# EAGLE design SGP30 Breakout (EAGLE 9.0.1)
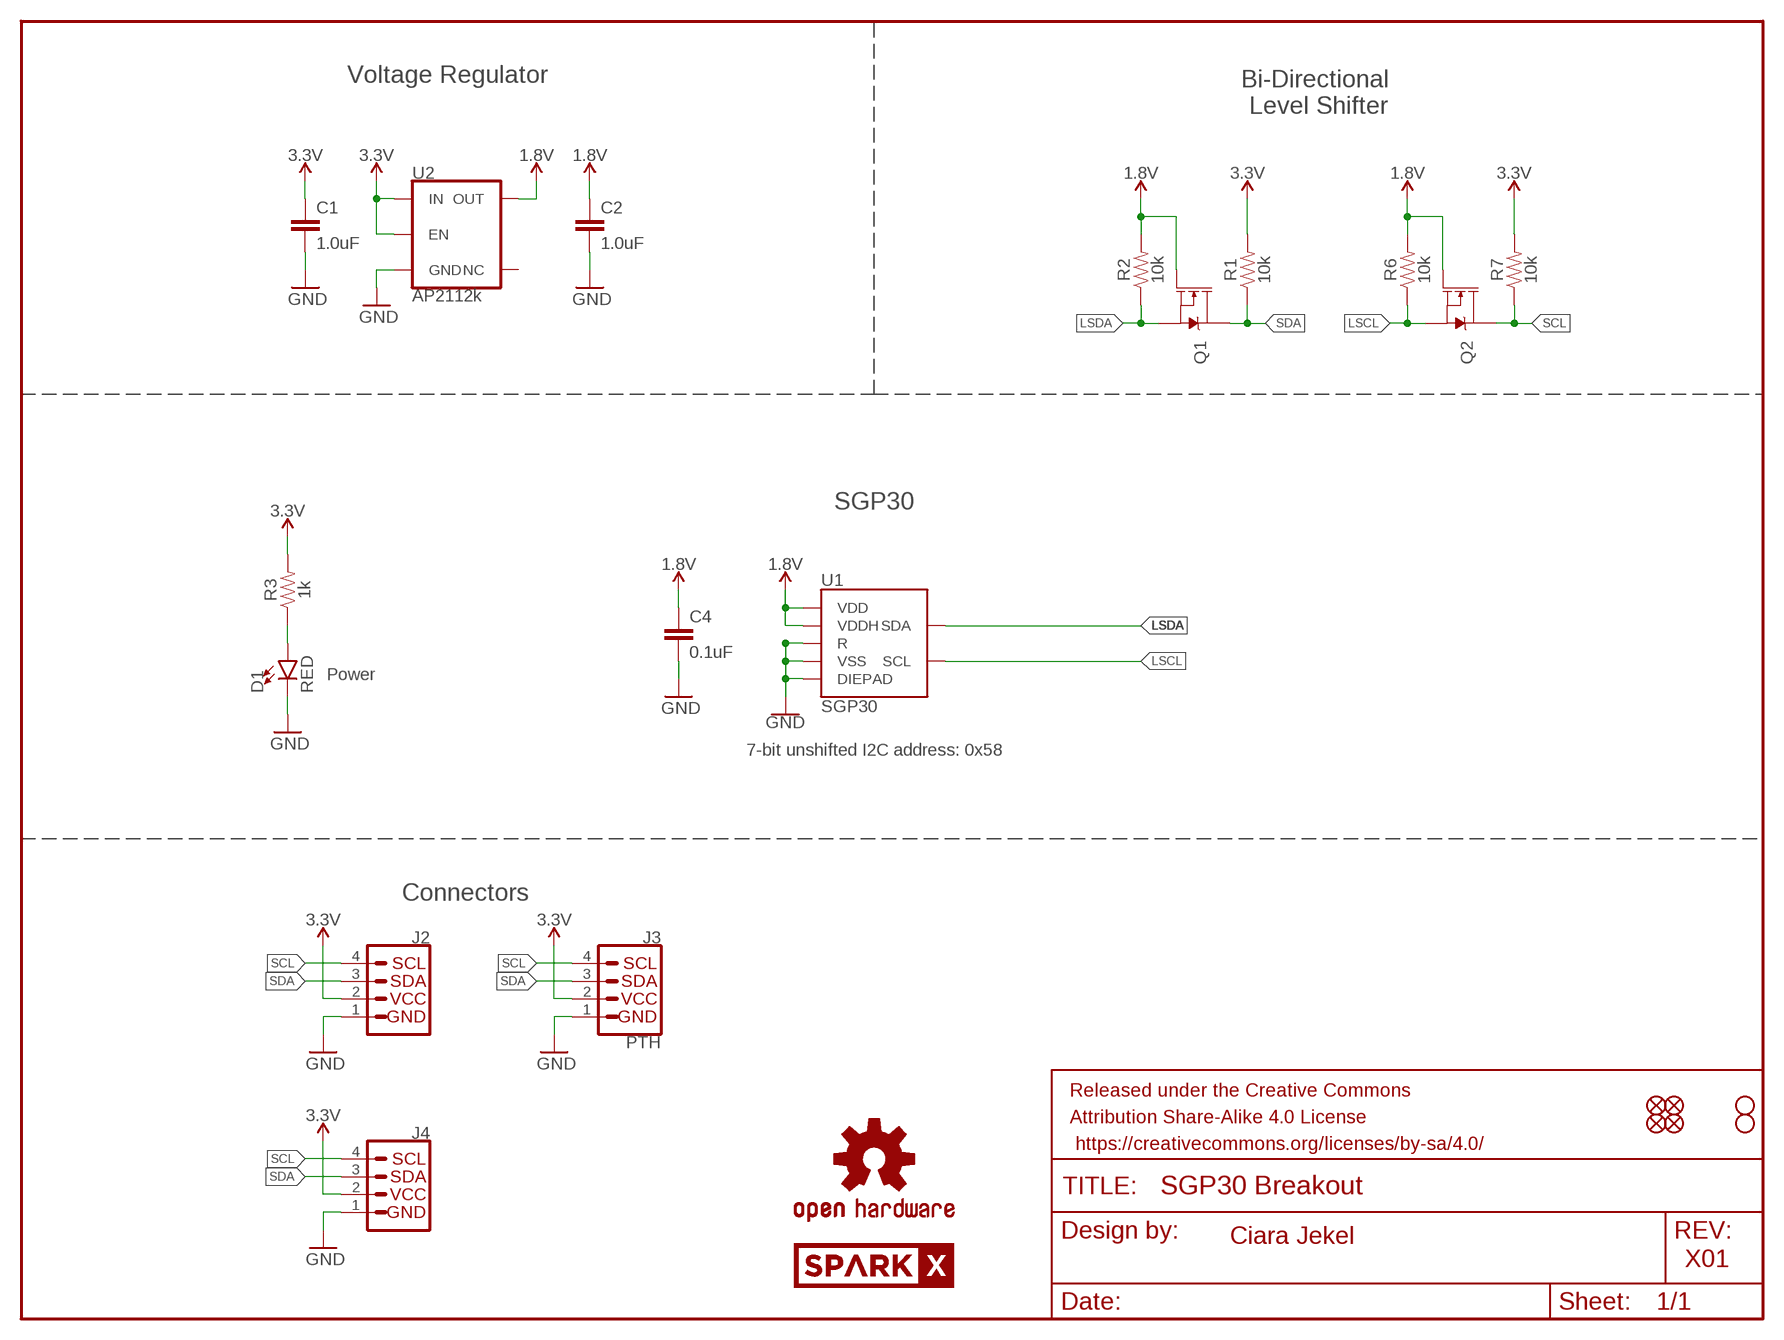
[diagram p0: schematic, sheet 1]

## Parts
C1  1.0uF  1.0UF-0603-16V-10%  [0603]
C2  1.0uF  1.0UF-0603-16V-10%  [0603]
C4  0.1uF  0.1UF-0603-25V-(+80/-20%)  [0603]
D1  RED  LED-RED0603  [LED-0603]
FRAME1  FRAME-LETTER  [CREATIVE_COMMONS]
J2  QWIIC_CONNECTORJS-1MM  [1X04_1MM_RA]
J3  PTH  I2C_STANDARD_NO_SILK  [1X04_NO_SILK]
J4  QWIIC_CONNECTORJS-1MM  [1X04_1MM_RA]
JP1  FIDUCIALUFIDUCIAL  [MICRO-FIDUCIAL]
JP2  FIDUCIALUFIDUCIAL  [MICRO-FIDUCIAL]
JP3  STAND-OFF  [STAND-OFF]
JP4  STAND-OFF  [STAND-OFF]
JP5  FIDUCIALUFIDUCIAL  [MICRO-FIDUCIAL]
JP6  FIDUCIALUFIDUCIAL  [MICRO-FIDUCIAL]
LOGO1  OSHW-LOGOMINI  [OSHW-LOGO-MINI]
Q1  MOSFET-NCH-BSS138  [SOT23-3]
Q2  MOSFET-NCH-BSS138  [SOT23-3]
R1  10k  10KOHM-0603-1/10W-1%  [0603]
R2  10k  10KOHM-0603-1/10W-1%  [0603]
R3  1k  1KOHM-0603-1/10W-1%  [0603]
R6  10k  10KOHM-0603-1/10W-1%  [0603]
R7  10k  10KOHM-0603-1/10W-1%  [0603]
U1  SGP30  [SGP30]
U2  AP2112k  MIC5504  [SOT23-5]
U$1  SPARKX-LOGO4  [SPARKX-MEDIUM]
U$2  SPARKX-LOGO4  [SPARKX-MEDIUM]

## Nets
1.8V: C2.1 C4.1 Q1.1(G) Q2.1(G) R2.2 R6.2 U1.1(VDD) U1.5(VDDH) U2.5(OUT)
3.3V: C1.1 J2.2 J3.2(VCC) J4.2 R1.2 R3.2 R7.2 U2.1(IN) U2.3(EN)
GND: C1.2 C2.2 C4.2 D1.C J2.1 J3.1(GND) J4.1 U1.2(VSS) U1.4(R) U1.DIEPAD U2.2(GND)
LSCL: Q2.2(S) R6.1 U1.6(SCL)
LSDA: Q1.2(S) R2.1 U1.3(SDA)
N$3: D1.A R3.1
SCL: J2.4 J3.4(SCL) J4.4 Q2.3(D) R7.1
SDA: J2.3 J3.3(SDA) J4.3 Q1.3(D) R1.1
Unconnected: U2.4(NC)

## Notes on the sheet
- Voltage Regulator
- Bi-Directional 
  Level Shifter
- SGP30
- Power
- 7-bit unshifted I2C address: 0x58
- Connectors
- Ciara Jekel
- X01

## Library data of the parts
C1 C2 = SparkFun-Capacitors:1.0UF: 1µF ceramic capacitors; PROD_ID: CAP-00868
C4 = SparkFun-Capacitors:0.1UF: 0.1µF ceramic capacitors; PROD_ID: CAP-00810
D1 = SparkFun-LED:LED-RED: Red SMD LED; PROD_ID: DIO-00819
FRAME1 = SparkFun-Aesthetics:FRAME-LETTER: Schematic Frame - Letter
J2 J4 = SparkFun-Connectors:QWIIC_CONNECTOR: SparkFun I2C Standard Qwiic Connector An SMD 1mm pitch JST connector makes it easy and quick (get it? Qwiic?) to connect I2C devices to each other. The Qwiic system enables fast and solderless connection between popular platforms and various sensors and actuators. We carry 200mm, 100mm, 50mm, and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; PROD_ID: CONN-13694
J3 = SparkX:I2C_STANDARD: SparkFun I2C Standard Pinout Header SparkFun has standardized on a pinout for all I2C based sensor breakouts. This pinout allows I2C boards to be plugged directly into the headers on Arduino Uno compatible boards, and to be daisy chained easily. Example SparkFun Products: SparkFun Atmospheric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
JP1 JP2 JP5 JP6 = SparkFun:FIDUCIAL: Fiducial Alignment Points
JP3 JP4 = SparkFun:STAND-OFF: Stand Off
LOGO1 = SparkFun-Aesthetics:OSHW-LOGO: Open-Source Hardware (OSHW) Logo
Q1 Q2 = SparkFun-DiscreteSemi:MOSFET-NCH: N-channel MOSFETs Voltage controlled devices that allow control of high current outputs. SparkFun Products: SparkFun OpenScale SparkFun Digital Sandbox SparkFun Monster Moto Shield SparkFun MOSFET Power Controller; PROD_ID: TRANS-00830; VALUE: 220mA/50V/3.5Ω
R1 R2 R6 R7 = SparkFun-Resistors:10KOHM: 10kΩ resistor; PROD_ID: RES-00824
R3 = SparkFun-Resistors:1KOHM: 1kΩ resistor; PROD_ID: RES-07856
U1 = SGP30:SGP30
U2 = SGP30:MIC5504
U$1 U$2 = SparkX:SPARKX-LOGO

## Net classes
1 power: width 0.203 mm

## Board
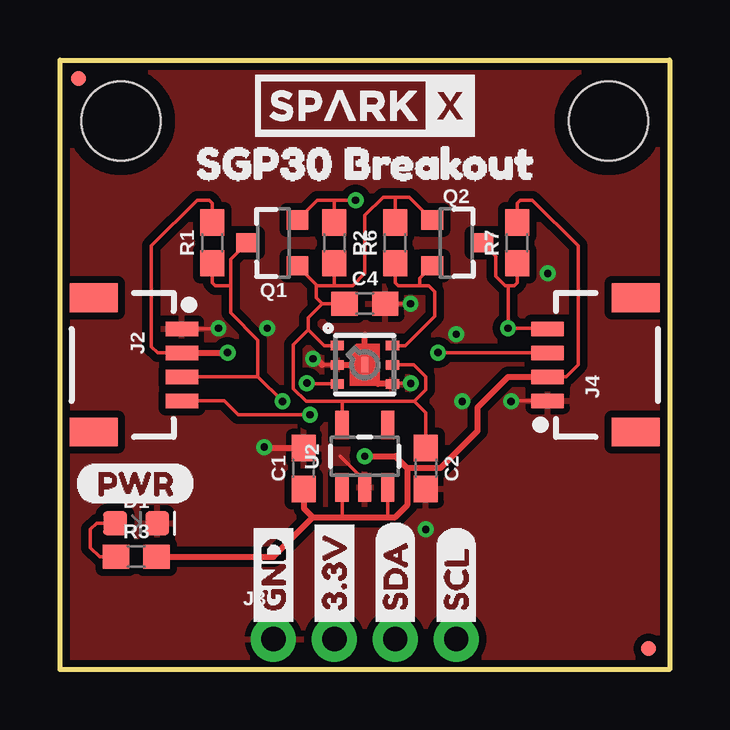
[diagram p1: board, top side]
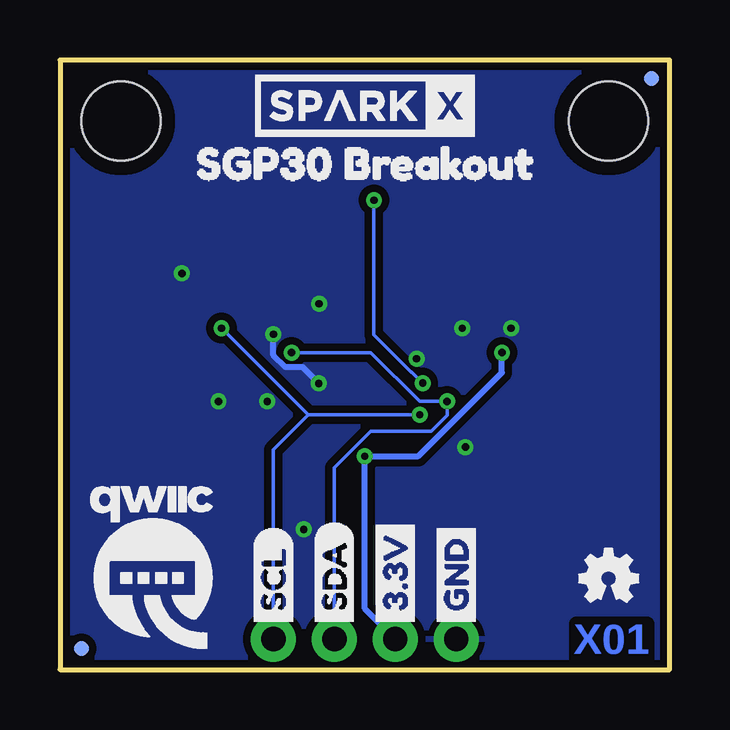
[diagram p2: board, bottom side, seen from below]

Size 25.4 x 25.4 mm. Coordinates in mm from the lower left corner, seen from the top.
Outline: 0,0 0,25.4 25.4,25.4 25.4,0 0,0
Copper layers (1*16): Top 0.035mm / dielectric 1.5mm / Bottom 0.035mm
Design rules "SparkFun-2-layer-PCBWay-LIMIT": minimum track width 6mil, minimum drill 0.3mm, track to track 6mil, track to pad 6mil, pad to pad 6mil, via to via 6mil, smd to smd 6mil, copper to edge 6mil, drill to drill 6mil, minimum pad ring 7mil, minimum via ring 7mil, stop-mask expansion 4mil, vias tented up to drill 25mil, thermal gap 10mil

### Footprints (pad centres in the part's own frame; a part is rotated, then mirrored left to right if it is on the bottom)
0603 = smd 1.1 x 1: 1 -0.85,0; 2 0.85,0
LED-0603 = smd 1 x 1: A -0.877,0; C 0.877,0
1X04_1MM_RA = smd 0.6 x 1.35: 1 -1.5,0; 2 -0.5,0; 3 0.5,0; 4 1.5,0 | smd 1.2 x 2: NC1 2.8,-3.675; NC2 -2.8,-3.675
1X04_NO_SILK = drill 1.016 pad 1.88: 1 0,0; 2 2.54,0; 3 5.08,0; 4 7.62,0
MICRO-FIDUCIAL = smd 0.635 x 0.635: 1 0,0
STAND-OFF = hole 3.302: 0,0
SOT23-3 = smd 0.8 x 0.9: 1 -0.95,-1; 2 0.95,-1; 3 0,1.1
SGP30 = smd 0.55 x 0.4: 1 -1.15,0.8; 2 -1.15,0; 3 -1.15,-0.8; 4 1.15,-0.8; 5 1.15,0; 6 1.15,0.8 | smd 0.305 x 0.61: DIEPAD 0,0
SOT23-5 = smd 0.55 x 1.2: 1 -0.95,-1.3; 2 0,-1.3; 3 0.95,-1.3; 4 0.95,1.3; 5 -0.95,1.3

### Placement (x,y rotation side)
C1  10.16,8.38 90 top
C2  15.24,8.38 270 top
C4  12.7,15.24 0 top
D1  3.17,6.1 0 top
FRAME1  not placed on the board
J2  5.08,12.7 270 top
J3  8.89,1.27 0 top
J4  20.32,12.7 90 top
JP1  0.76,24.64 0 bottom
JP2  24.51,0.89 0 top
JP3  2.54,22.86 0 top
JP4  22.86,22.86 0 top
JP5  24.51,0.89 0 bottom
JP6  0.76,24.64 0 top
LOGO1  2.54,3.81 0 bottom
Q1  8.89,17.78 90 top
Q2  16.51,17.78 270 top
R1  6.35,17.78 90 top
R2  11.43,17.78 270 top
R3  3.17,4.7 0 top
R6  13.97,17.78 90 top
R7  19.05,17.78 90 top
U1  12.7,12.7 0 top
U2  12.7,8.89 0 top
U$1  12.7,23.5 0 top
U$2  12.7,23.5 0 bottom
U$3  [GND1]  8.89,1.52 90 bottom
U$4  [3#3V2]  11.43,1.52 90 bottom
U$5  [SDA8]  13.97,1.52 90 bottom
U$6  [SCL9]  16.51,1.52 90 bottom
U$7  [SGP30_BREAKOUT1]  4.57,21.08 0 top
U$8  [SGP30_BREAKOUT1]  20.83,21.08 0 bottom
U$10  [(PWR)]  0.64,7.75 0 top
U$21  [3#3V2]  11.43,1.52 90 top
U$22  [GND1]  8.89,1.52 90 top
U$26  [SCL9]  16.51,1.52 90 top
U$27  [SDA8]  13.97,1.52 90 top
U$29  [QWIIC-LOGO-MEDIUM]  21.59,4.32 0 bottom

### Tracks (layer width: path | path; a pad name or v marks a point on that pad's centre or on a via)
1.8V
  Top 0.152: 10.92,15.24 C4.1 | U1.5 14.73,12.7 15.24,12.19 15.24,11.66 14.76,11.18 | 10.35,14.16 11.01,13.5 U1.1 | 10.35,14.16 9.73,13.54 9.73,11.71 10.26,11.18 11.75,11.18 | 14.76,11.18 11.75,11.18 | U2.5 11.75,11.18 | 10.35,14.16 10.35,14.67 10.92,15.24 | 10.92,15.24 10.67,15.49 10.67,16 10.72,16 | 13.97,19.68 13.46,19.68 12.7,18.92 12.7,16.51 12.19,16 11.43,16 | R2.2 11.43,16 | R6.2 13.97,19.68 | C2.1 15.24,10.7 14.76,11.18 | Q2.1 14.55,19.68 13.97,19.68 | Q1.1 10.72,16 | 10.72,16 11.43,16
3.3V  (via drill 0.3)
  Top 0.152: 11.68,6.35 13.65,6.35 | 13.65,6.35 13.97,6.35 | U2.3 13.65,6.35 | R7.2 19.05,19.43 19.18,19.56 19.68,19.56 21.59,17.65 21.59,12.7 21.09,12.2 J4.2 20.19,12.2 20.2,12.19 | R1.2 6.35,19.43 6.22,19.56 5.71,19.56 3.81,17.65 3.81,13.46 4.07,13.2 J2.2 | 10.54,6.35 11.68,6.35 | 11.68,6.35 11.75,6.42 U2.1
  Top 0.254: J2.2 v6.99,13.21 | v12.7,8.89 13.97,8.89 14.46,8.4 | 20.19,12.2 18.67,12.2 17.4,10.93 17.4,9.95 15.86,8.4 14.46,8.4 | R3.2 8.89,4.7 10.54,6.35 | C1.1 10.16,6.73 10.54,6.35 | 10.54,6.35 13.97,6.35 14.46,6.84 14.46,8.4
  Bottom 0.254: v6.99,13.21 6.99,12.37 10.47,8.89 v12.7,8.89 12.7,2.54 J3.2
GND  (via drill 0.3)
  Top 0.152: 10.92,12.7 U1.2 12.45,12.7 | C4.2 v14.61,15.24 | J2.1 6.58,14.2 v6.6,14.22 | J4.1 18.82,11.2 v18.8,11.18 | U1.4 13.88,11.93 v14.62,11.93 | 12.45,12.7 12.57,12.7 | 13.21,11.94 12.45,12.7 | U2.2 12.7,7.87 11.68,8.89
  Top 0.254: v10.54,12.95 10.67,12.95 10.92,12.7 | C1.2 8.55,9.23 v8.51,9.27 | U1.2 12.57,12.7 | 12.57,12.7 U1.DIEPAD 12.7,13.97 | U1.4 13.25,11.9 13.21,11.94 12.57,12.57 12.57,12.7
  Bottom 0.254: v14.62,11.93 15.29,12.6 16,12.6 16.51,13.11 v16.51,13.97
  other vias: 8.64,14.22 15.24,5.84 16.76,11.18 20.32,16.51
  pour Bottom (isolate 0.305): 0,0 0,25.4 25.4,25.4 25.4,0
  pour Top (isolate 0.305): 0,0 0,25.4 25.4,25.4 25.4,0
LSCL
  Top 0.152: U1.6 14.39,13.5 15.62,14.73 15.62,15.75 15.37,16 14.99,16 | R6.1 13.97,16.13 14.1,16 14.99,16 | Q2.2 14.99,16.31 14.99,16
LSDA  (via drill 0.3)
  Top 0.152: 11.43,19.56 v12.32,19.56 | R2.1 11.43,19.56 | U1.3 10.32,11.9 v10.29,11.94 | Q1.2 10.72,19.56 11.43,19.56
  Bottom 0.152: 10.16,12.06 v10.29,11.94 10.74,12.39 10.77,12.39 12.32,13.94 v12.32,19.56
N$3
  Top 0.152: R3.1 1.65,4.7 1.27,5.08 1.27,5.84 1.52,6.1 D1.A
SCL  (via drill 0.3)
  Top 0.152: 20.32,14.22 J4.4 20.3,14.22 v18.67,14.22 18.67,16 | 5.1,11.18 J2.4 6.83,11.2 7.42,10.62 v10.41,10.62 | Q2.3 18.16,17.23 18.16,16.38 18.54,16 18.67,16 | 18.67,16 18.92,16 19.05,16.13 R7.1
  Bottom 0.152: v18.67,14.22 15.06,10.62 | 15.06,10.62 v10.41,10.62 | J3.4 16.51,9.17 15.06,10.62
SDA  (via drill 0.3)
  Top 0.152: J4.3 v15.76,13.2 v15.75,13.21 | v9.27,11.18 8.25,12.2 | 8.25,12.2 J2.3 | 8.25,12.2 8.25,13.72 7.11,14.86 7.11,16 | R1.1 6.35,16.13 6.48,16 7.11,16 | Q1.3 7.11,17.1 7.11,16
  Bottom 0.152: v15.75,13.21 12.45,13.21 10.41,11.18 v9.27,11.18 9.27,10.59 9.93,9.93 12.45,9.93 13.97,8.41 J3.3

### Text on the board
Bottom: X01
Measures: Dimensions in inches
tDocu: Ciara Jekel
